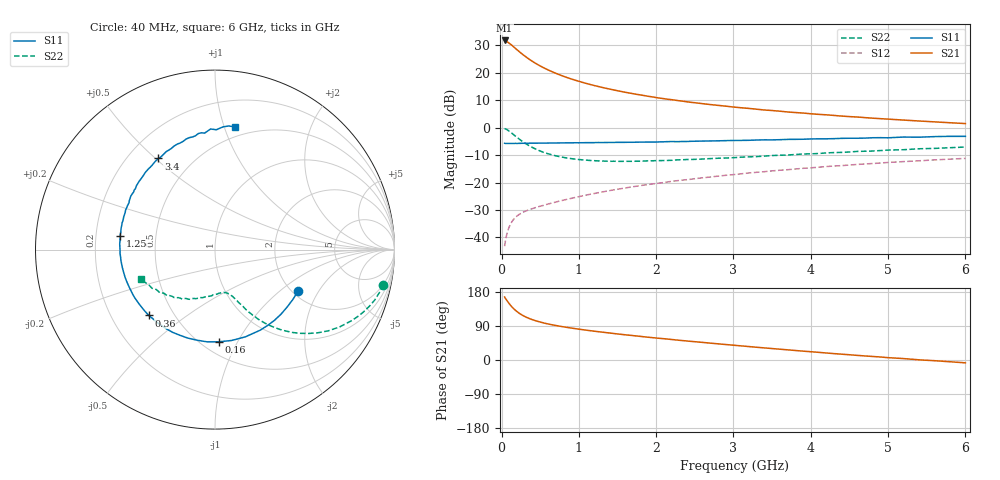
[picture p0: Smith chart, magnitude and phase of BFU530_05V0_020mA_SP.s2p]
! Filename:  P:\Prog\Test\Noise\ATS_data\Testdata_Net\03 Spar\BFU530_APG2013_40_A05_05p0V_020mA_SP_CM01_D.s2p
! Date/Time: Fri 26/Apr/2013 13:03:14
! BFU530_APG2013_40_A05_05p0V_1to25mA_SP_CM01_Bias7_R.s2p
! MDIF S-parameter v. bias file
! BFU530_APG2013_40_A05_05p0V_1to25mA_SP_CM01
! Date/time Wed Apr 24 19:36:53 2013
! VAR V_out= 5.0000
! VAR I_out= 20.0000
! VAR V_in= 0.8382
! VAR I_in= 0.2230
! Device data file deembeded for feedlines and parallel
! Original file: \03 Spar\BFU530_APG2013_40_A05_05p0V_020mA_SP_CM01_R.s2p
! Feed-files: PR047V01_250413_Feed1.s2p, PR047V01_250413_Feed2.s2p
! Parallel-file: PR047V01_250413_Par.s2p
# MHz S MA R 50
!  Freq-MHz  S11-mag  S11-arg  S21-mag  S21-arg  S12-mag  S12-arg  S22-mag  S22-arg
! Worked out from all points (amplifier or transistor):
!   98 points, 40 MHz to 6 GHz, reference 50 ohm
!   highest |S21| = 31.7 dB at 40 MHz (marker M1)
!   |S21| within 3 dB of that: start of sweep to 184.5 MHz
!   unconditionally stable (mu >= 1): 1.276 GHz to 3.474 GHz
!   at 300 MHz: K = 0.48, MSG = 28.3 dB, |S12| = -30.5 dB
!   at 1.6 GHz: K = 1.04, MAG = 16.2 dB, |S12| = -22.0 dB
!   at 6 GHz: K = 0.86, MSG = 6.3 dB, |S12| = -11.2 dB
!   S11 on the Smith chart (normalised r, x): 40 MHz: 2.16, -1.35; 160 MHz: 0.60, -0.84; 360 MHz: 0.36, -0.36; 1.25 GHz: 0.30, +0.07; 3.4 GHz: 0.32, +0.51; 6 GHz: 0.41, +1.09
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40  0.5174 -26.2  38.49 166.3  0.006951 80.3  0.9589 -11.8
50  0.5152 -32.6  38.19 162.5  0.008561 78.2  0.9473 -14.6
90  0.5144 -55.7  34.99 151.2  0.01438 69.9  0.8784 -25.1
120  0.5147 -70.9  32.59 143.5  0.01791 65.0  0.8173 -31.8
140  0.5147 -79.7  30.89 139.0  0.01989 62.3  0.7766 -35.6
160  0.5141 -87.6  29.16 134.9  0.02168 59.9  0.7373 -39.0
200  0.5146 -101.2  26.08 127.8  0.02458 56.4  0.6636 -44.6
240  0.5158 -112.3  23.41 121.9  0.02689 54.1  0.6009 -49.0
300  0.5176 -125.3  20.09 114.9  0.02976 52.0  0.5252 -53.9
360  0.5202 -135.2  17.46 109.5  0.03213 51.1  0.467 -57.5
460  0.5208 -147.3  14.22 102.5  0.03575 51.2  0.3969 -61.5
600  0.5227 -159.3  11.25 95.2  0.04057 52.5  0.3347 -65.0
800  0.5263 -170.8  8.596 87.6  0.04777 54.6  0.2872 -68.7
1050  0.5304 178.2  6.629 80.0  0.05726 56.6  0.2588 -72.7
1250  0.5343 171.6  5.599 74.8  0.06524 57.7  0.2474 -75.7
1600  0.5391 161.0  4.389 66.5  0.07951 58.1  0.2435 -82.0
2050  0.5493 150.5  3.434 57.1  0.09807 57.5  0.2506 -90.3
3100  0.5841 127.9  2.294 37.2  0.1442 53.1  0.2893 -110.0
3400  0.5976 121.9  2.09 31.9  0.1575 51.1  0.3026 -115.5
4100  0.6243 109.6  1.74 20.2  0.1898 46.1  0.3373 -127.6
5200  0.6724 92.1  1.369 3.8  0.2403 37.0  0.3956 -145.8
6000  0.6926 80.8  1.183 -7.5  0.275 29.4  0.4426 -158.4
